PROGRAM Tc2_DALI_Test
VAR
	nStep				:	INT;
	fbTon				:	TON;
	fbOff				:	FB_DALIV2Off();
	fbGetEventData		:	FB_DALIV2GetEventData();
	nRisingEdge			:	INT;
	nFallingEdge		:	INT;
END_VAR

CASE nStep OF
0:
	fbTon(IN := TRUE, PT := T#1S);		
	IF (fbTon.Q) THEN
		fbTon(IN := FALSE);
		fbOff(bStart := FALSE, stCommandBuffer := GVL.stCommandBufferKL6821);
		nStep := 10;
	END_IF

10:
	fbOff(	bStart := TRUE,
			nAddr := 0,
			stCommandBuffer := GVL.stCommandBufferKL6821);
	IF (NOT fbOff.bBusy) THEN
		fbOff(bStart := FALSE, stCommandBuffer := GVL.stCommandBufferKL6821);
		nStep := 0;
	END_IF
ELSE
	fbOff(bStart := FALSE, stCommandBuffer := GVL.stCommandBufferKL6821);
	fbTon(IN := FALSE);
	nStep := 0;
END_CASE

fbGetEventData(	bEnable := TRUE,
				eEventScheme := eDALIV2EventSchemeDeviceInstance,
				nAddressInfo01 := 3,
				nAddressInfo02 := 0,
				stCommandBuffer := GVL.stCommandBufferKL6821);
IF (fbGetEventData.bNewData) THEN
	IF (fbGetEventData.nEventInfo = 16#0001) THEN // Button pushed		
		nRisingEdge := nRisingEdge + 1;
	END_IF
	IF (fbGetEventData.nEventInfo = 16#0000) THEN // Button released
		nFallingEdge := nFallingEdge + 1;
	END_IF
END_IF

END_PROGRAM
